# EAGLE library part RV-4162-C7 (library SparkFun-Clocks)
[RV-4162-C7] - [Real Time Clock Module with I2C Bus] Specifications: Pin count: [8] Pin pitch: [.9mm] Area: [3.2mm x 1.5mm] Datasheet referenced for footprint Example device(s): [EXAMPLE DEVICE 1] [EXAMPLE DEVICE 2]
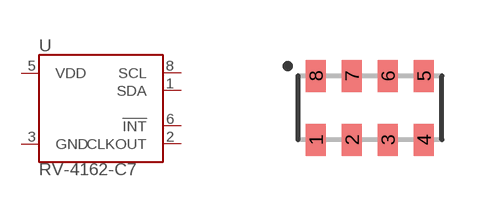
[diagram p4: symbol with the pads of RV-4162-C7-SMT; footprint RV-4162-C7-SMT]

Designator prefix U

## RV-4162-C7 (PROD_ID: IC-13900)  [RV-4162-C7-SMT]
1  SDA
2  CLKOUT
3  GND
5  VDD
6  !INT
8  SCL

## Footprint RV-4162-C7-SMT (pad centres in mm)
smd 0.5 x 0.8: 1 -1.35,-0.8; 2 -0.45,-0.8; 3 0.45,-0.8; 4 1.35,-0.8; 5 1.35,0.8; 6 0.45,0.8; 7 -0.45,0.8; 8 -1.35,0.8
